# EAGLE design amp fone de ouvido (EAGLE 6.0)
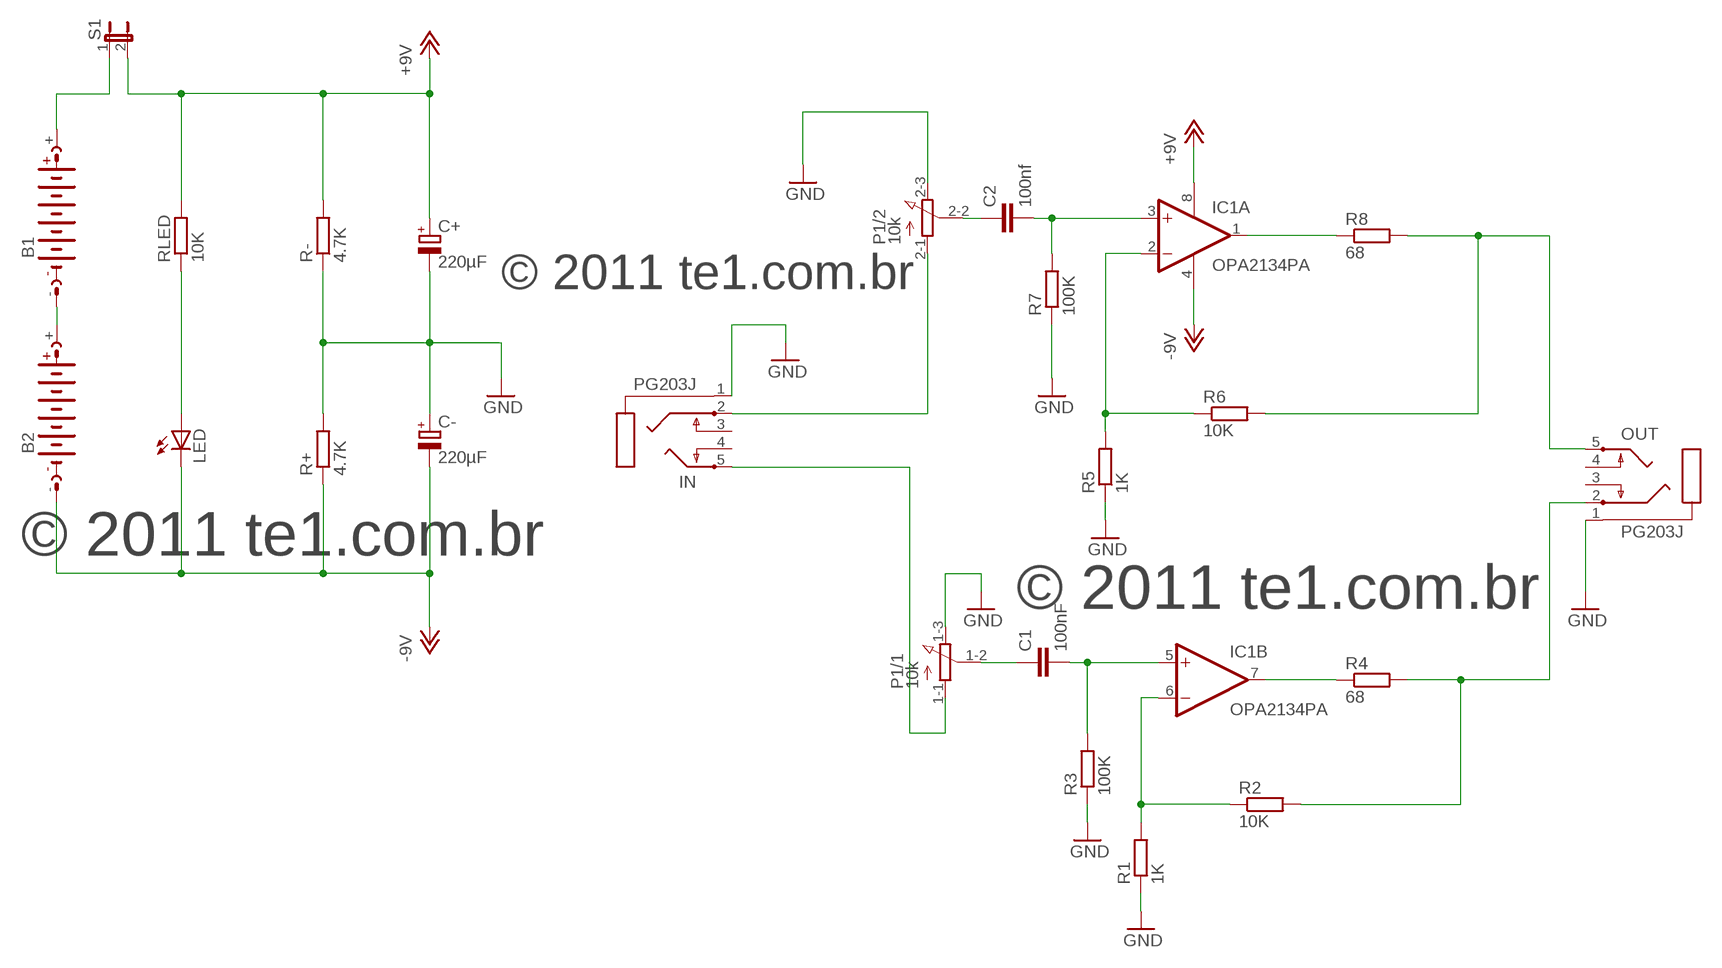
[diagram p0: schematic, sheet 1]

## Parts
B1  AB9V  [AB9V]
B2  AB9V  [AB9V]
C1  100nF  C7.5/3  [C7.5B3]
C2  100nf  C7.5/3  [C7.5B3]
C+  220µF  CPOL-EUE3.5-8  [E3,5-8]
C-  220µF  CPOL-EUE3.5-8  [E3,5-8]
IC1  OPA2134PA  [DIL08]
IN  PG203J  [PG203J]
LED  LED3MM  [LED3MM]
OUT  PG203J  [PG203J]
P1  10k  3RP/1610G  [3RP/1610G]
R1  1K  R-EU_0207/7  [0207/7]
R2  10K  R-EU_0207/7  [0207/7]
R3  100K  R-EU_0207/7  [0207/7]
R4  68  R-EU_0207/7  [0207/7]
R5  1K  R-EU_0207/2V  [0207/2V]
R6  10K  R-EU_0207/7  [0207/7]
R7  100K  R-EU_0207/7  [0207/7]
R8  68  R-EU_0207/7  [0207/7]
R+  4.7K  R-EU_0207/7  [0207/7]
R-  4.7K  R-EU_0207/7  [0207/7]
RLED  10K  R-EU_0207/7  [0207/7]
S1  JP1E  [JP1]

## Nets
+12V: C+.+ IC1.8(A:V+) R-.2 RLED.2 S1.2 ; supply symbol labelled +9V
-12V: B2.- C-.- IC1.4(A:V-) LED.K(C) R+.1 ; supply symbol labelled -9V
GND: C+.- C-.+ IN.1 OUT.1 P1.1-3(/1:E) P1.2-3(/2:E) R1.1 R3.1 R5.1 R7.1 R+.2 R-.1
N$1: B1.- B2.+
N$2: C2.2 IC1.3(A:+IN) R7.2
N$3: LED.A RLED.1
N$4: C2.1 P1.2-2(/2:S)
N$5: IC1.1(A:OUT) R8.1
N$6: C1.2 IC1.5(B:+IN) R3.2
N$7: OUT.5 R6.2 R8.2
N$8: IC1.2(A:-IN) R5.2 R6.1
N$9: IC1.6(B:-IN) R1.2 R2.1
N$10: IC1.7(B:OUT) R4.1
N$11: IN.2 P1.2-1(/2:A)
N$12: IN.5 P1.1-1(/1:A)
N$15: B1.+ S1.1
N$16: C1.1 P1.1-2(/1:S)
N$17: OUT.2 R2.2 R4.2
Unconnected: IN.3 IN.4 OUT.3 OUT.4

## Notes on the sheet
- © 2011 te1.com.br
- © 2011 te1.com.br
- © 2011 te1.com.br

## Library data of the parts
B1 B2 = battery:AB9V: 9-V BATTERY CLIP
C1 C2 = capacitor-wima:C: CAPACITOR
C+ C- = rcl:CPOL-EU: POLARIZED CAPACITOR, European symbol
IC1 = linear:OPA2*: Dual Operational Amplifier Low Power, Single-Supply, Rail-To-Rail Operational Amplifier Source: http://focus.ti.com/lit/ds/symlink/opa2345.pdf http://focus.ti.com .. opa241.pdf http://focus.ti.com/lit/ds/symlink/opa2134.pdf
IN OUT = con-hirschmann:PG203J: MIC/HEADPHONE JACK KS-S stereo microphone/headphone jack PG203JN (Schukat); OC_FARNELL: unknown; OC_NEWARK: unknown
LED = led:LED: LED
P1 = pot:3RP/1610G: 16mm Potentiometer two level Source: http://www.alphapotentiometers.net/html/16mm_pot_2.html
R1-R8 R+ R- RLED = rcl:R-EU_: RESISTOR, European symbol
S1 = jumper:JP1E: JUMPER

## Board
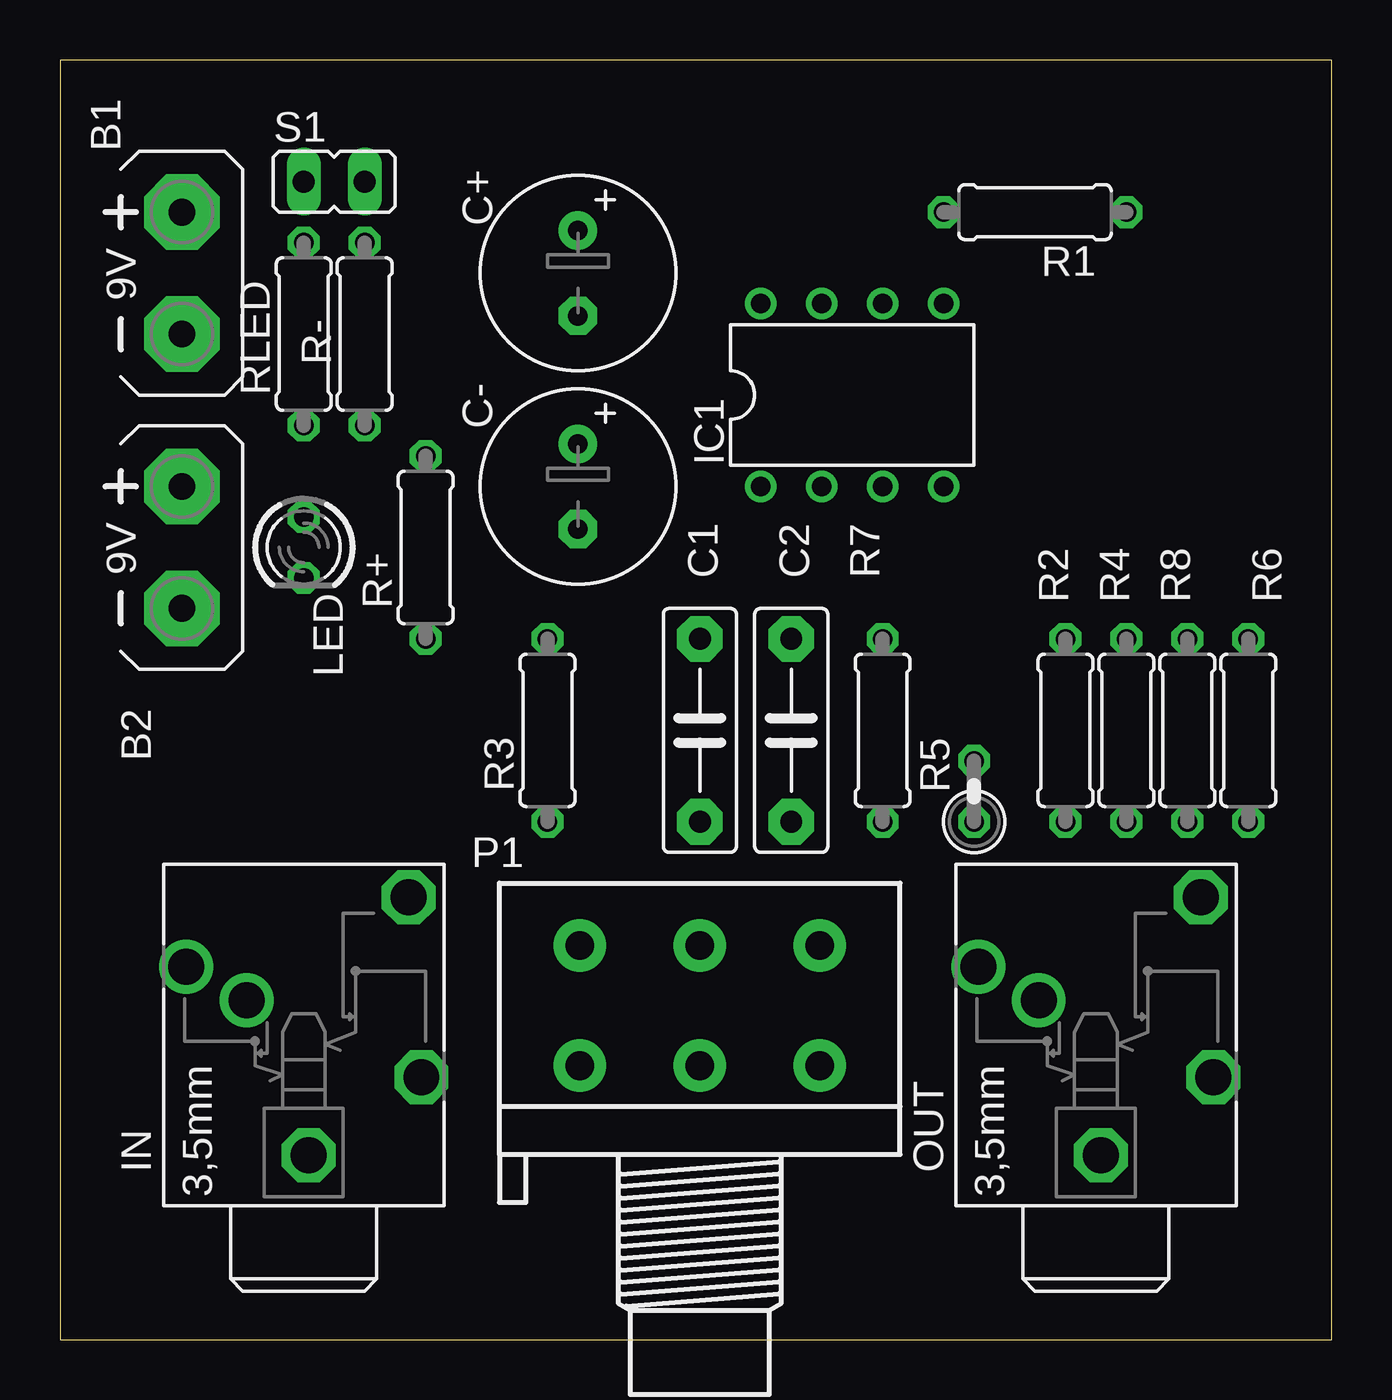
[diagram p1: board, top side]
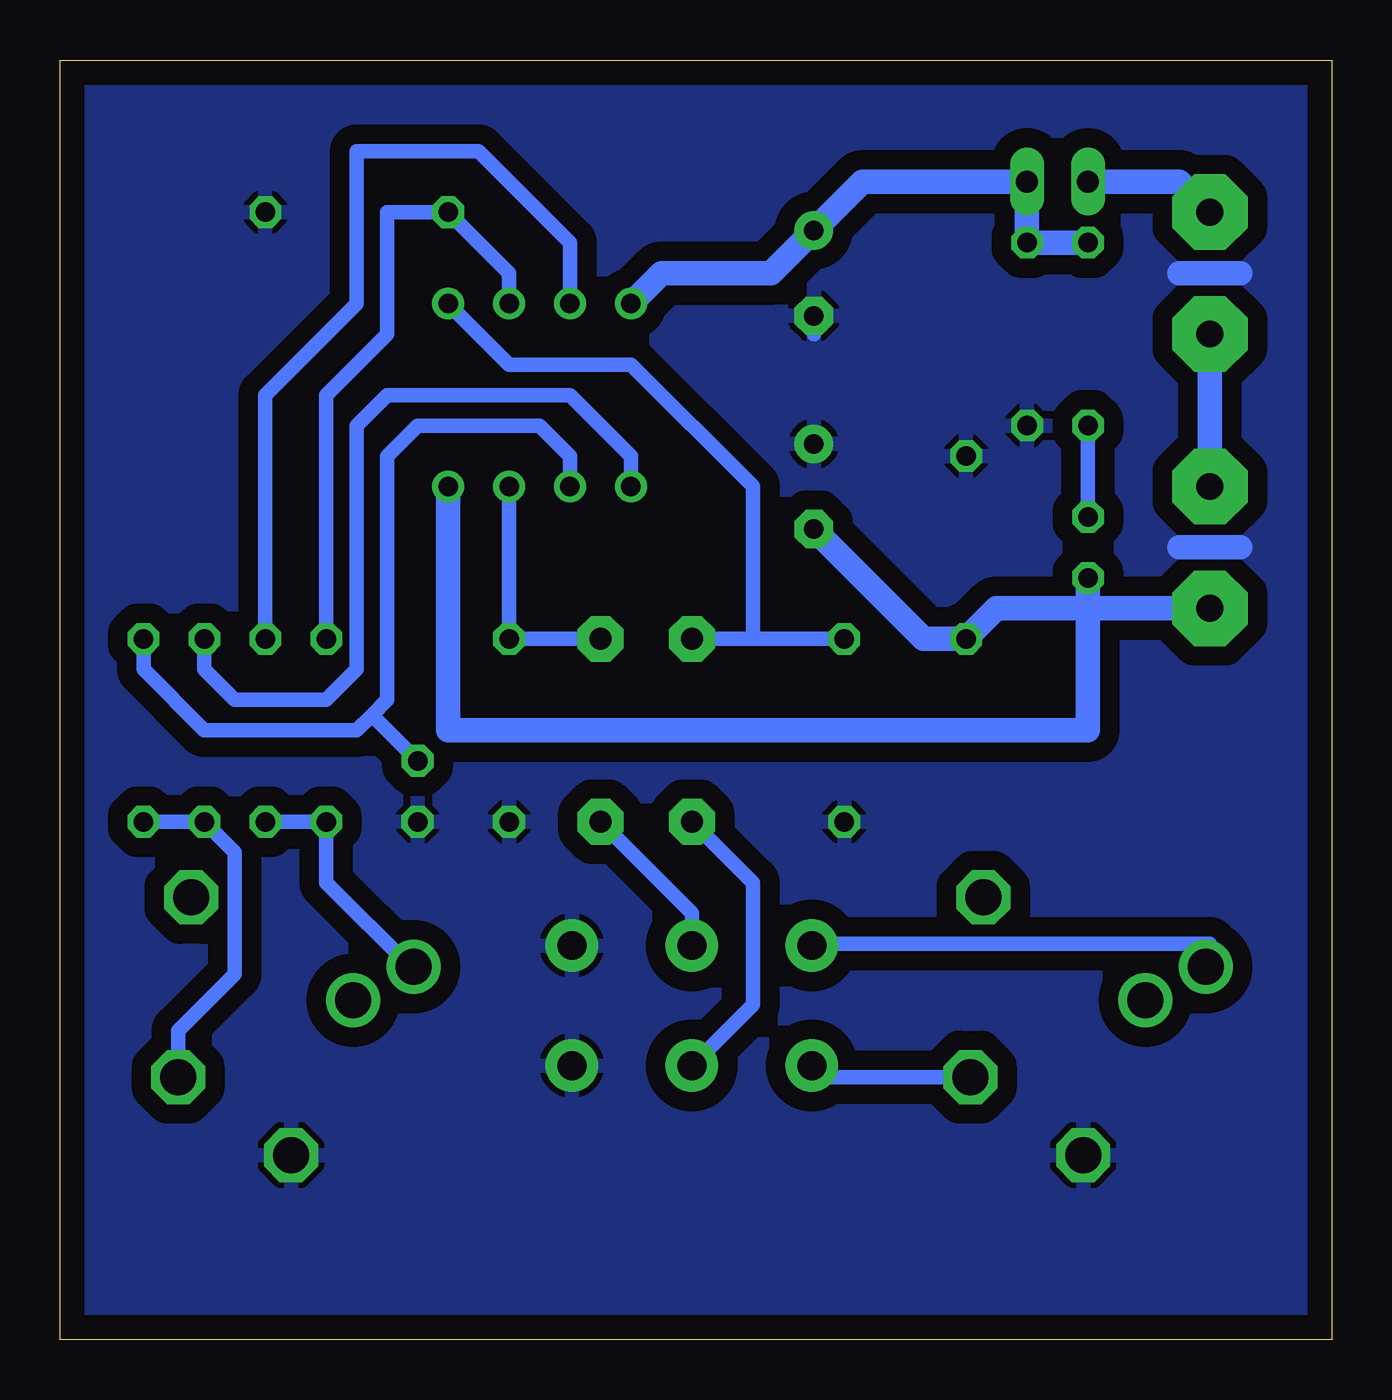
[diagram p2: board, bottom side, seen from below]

Size 53.01 x 53.33 mm. Coordinates in mm from the lower left corner, seen from the top.
Outline: 0,0 53.01,0 53.01,53.33 0,53.33 0,0
Copper layers (1*16): Top 0.035mm / dielectric 1.5mm / Bottom 0.035mm
Design rules: minimum track width 10mil, minimum drill 24mil, track to track 8mil, track to pad 8mil, pad to pad 8mil, via to via 8mil, smd to smd 8mil, copper to edge 40mil, drill to drill 8mil, minimum pad ring 10mil, minimum via ring 8mil, stop-mask expansion 4mil, vias tented up to drill 0mil, thermal gap 10mil

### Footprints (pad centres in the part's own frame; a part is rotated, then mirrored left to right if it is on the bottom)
AB9V = drill 1.118 pad 3.15 octagon: + 0,2.54; - 0,-2.54
C7.5B3 = drill 0.914 pad 1.905 octagon: 1 -3.81,0; 2 3.81,0
E3,5-8 = drill 0.813 pad 1.6: + -1.778,0 | drill 0.813 pad 1.6 octagon: - 1.778,0
DIL08 = drill 0.813 pad 1.27: 1 -3.81,-3.81; 2 -1.27,-3.81; 3 1.27,-3.81; 4 3.81,-3.81; 5 3.81,3.81; 6 1.27,3.81; 7 -1.27,3.81; 8 -3.81,3.81
PG203J = drill 1.499 octagon: 1 -5.004,-0.203; 4 5.74,-4.369; 5 -1.753,-4.902 | drill 1.499: 2 2.845,4.902; 3 1.448,2.388
LED3MM = drill 0.813 octagon: A -1.27,0; K 1.27,0
3RP/1610G = drill 1.2 pad 2.184: 1-1 -5,0; 1-2 0,0; 1-3 5,0; 2-1 -5,5; 2-2 0,5; 2-3 5,5
0207/7 = drill 0.813 octagon: 1 -3.81,0; 2 3.81,0
0207/2V = drill 0.813 octagon: 1 -1.27,0; 2 1.27,0
JP1 = drill 0.914 long: 1 0,-1.27; 2 0,1.27

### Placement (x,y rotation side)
B1  5.08,44.45 0 top
B2  5.08,33.02 0 top
C1  26.67,25.4 90 top
C2  30.48,25.4 90 top
C+  21.59,44.45 270 top
C-  21.59,35.56 270 top
IC1  33.02,39.37 0 top
IN  10.16,12.7 90 top
LED  10.16,33.02 270 top
OUT  43.18,12.7 90 top
P1  26.67,11.43 0 top
R1  40.64,46.99 180 top
R2  41.91,25.4 270 top
R3  20.32,25.4 90 top
R4  44.45,25.4 270 top
R5  38.1,22.86 90 top
R6  49.53,25.4 270 top
R7  34.29,25.4 90 top
R8  46.99,25.4 270 top
R+  15.24,33.02 90 top
R-  12.7,41.91 90 top
RLED  10.16,41.91 90 top
S1  11.43,48.26 270 top

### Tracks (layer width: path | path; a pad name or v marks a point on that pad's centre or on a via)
+12V
  Bottom 1.016: IC1.8 27.94,44.45 23.37,44.45 C+.+ 19.56,48.26 S1.2 R-.2 RLED.2
-12V
  Bottom 1.016: 10.16,30.48 10.16,25.4 36.83,25.4 IC1.4 | 10.16,30.48 LED.K | B2.- 10.16,30.48 | 10.16,30.48 13.97,30.48 R+.1 17.02,29.21 C-.-
GND
  Bottom 0.61: 21.59,41.91 C+.- 21.59,43.18
  Bottom 1.016: 3.81,33.02 6.35,33.02 | 3.81,44.45 6.35,44.45
  pour Bottom (isolate 0.813): 0,53.34 0,0 53.34,0 53.34,53.34
N$1
  Bottom 1.016: B1.- B2.+
N$2
  Bottom 0.61: C2.2 R7.2 IC1.3
N$3
  Bottom 0.61: LED.A RLED.1
N$4
  Bottom 0.61: P1.2-2 26.67,17.78 C2.1
N$5
  Bottom 0.61: IC1.1 29.21,36.83 31.75,39.37 39.37,39.37 40.64,38.1 40.64,27.94 41.91,26.67 45.72,26.67 46.99,27.94 R8.1
N$6
  Bottom 0.61: C1.2 24.13,29.21 | 24.13,29.21 R3.2 | IC1.5 34.29,40.64 29.21,40.64 24.13,35.56 24.13,29.21
N$7
  Bottom 0.61: OUT.5 48.08,12.88 45.72,15.24 45.72,20.32 R8.2 R6.2
N$8
  Bottom 0.61: IC1.2 31.75,36.83 33.02,38.1 38.1,38.1 39.37,36.83 39.37,26.67 40.01,26.04 | 40.01,26.04 40.64,25.4 46.99,25.4 49.53,27.94 R6.1 | R5.2 40.01,26.04
N$9
  Bottom 0.61: IC1.6 34.29,44.45 R1.2 39.37,46.99 39.37,41.91 41.91,39.37 R2.1
N$10
  Bottom 0.61: IC1.7 31.75,45.72 35.56,49.53 40.64,49.53 40.64,43.18 44.45,39.37 R4.1
N$11
  Bottom 0.61: IN.2 5.26,16.33 5.08,16.51 21.59,16.51 P1.2-1
N$12
  Bottom 0.61: IN.5 21.19,10.95 P1.1-1
N$15
  Bottom 1.016: B1.+ 6.35,48.26 S1.1
N$16
  Bottom 0.61: C1.1 24.13,19.05 24.13,13.97 P1.1-2
N$17
  Bottom 0.61: OUT.2 38.41,15.54 41.91,19.05 R2.2 R4.2

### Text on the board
Holes: © 2011 te1.com.br | © 2011 te1.com.br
